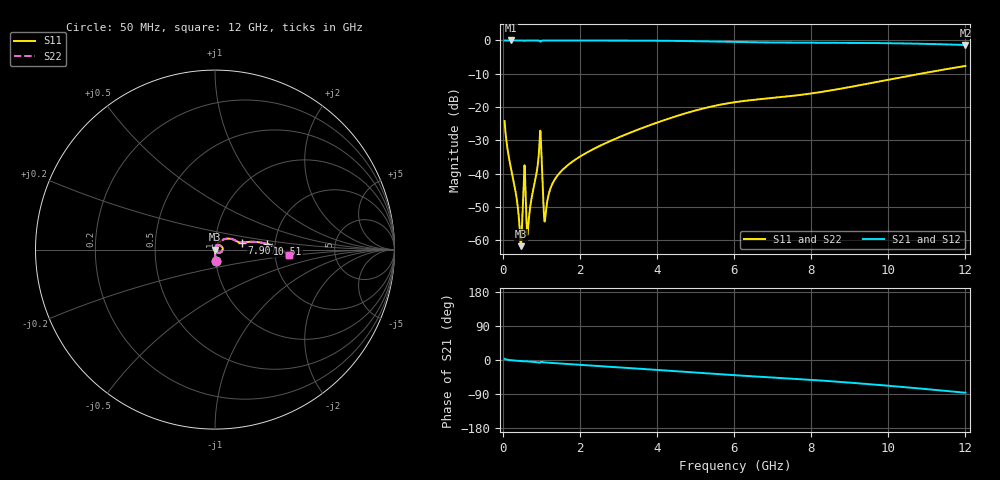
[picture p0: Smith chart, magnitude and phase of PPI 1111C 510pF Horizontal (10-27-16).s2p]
# MHz S MA R 50
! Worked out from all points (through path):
!   1601 points, 50 MHz to 12 GHz, reference 50 ohm
!   highest |S21| = 0.00 dB at 214.3 MHz (marker M1); lowest = -1.4 dB at 12 GHz (marker M2)
!   group delay of S21, straight-line fit = 19.5 ps
!   lowest |S11| = -61.8 dB at 475.7 MHz (marker M3), VSWR 1.00, Z = 50.1 + j0.00375 ohm
!   |S11| at or under -10 dB: start of sweep to 10.84 GHz
!   |S22| runs from -61.8 to -7.7 dB; largest |S21 - S12| = 0
!   S11 on the Smith chart (normalised r, x): 50 MHz: 1.00, -0.12; 7.907 GHz: 1.35, +0.11; 10.51 GHz: 1.81, +0.12; 12 GHz: 2.39, -0.19
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50  0.06142 -86.5  0.9978 3.2  0.9978 3.2  0.06142 -86.5
214.3125  0.01205 -88.3  0.9994 -0.6  0.9994 -0.6  0.01205 -88.3
348.75  0.00476 -84.8  0.9994 -1.8  0.9994 -1.8  0.00476 -84.8
430.9062  0.001803 -70.2  0.9993 -2.4  0.9993 -2.4  0.001803 -70.2
475.7188  0.0008118 2.6  0.9992 -2.8  0.9992 -2.8  0.0008118 2.6
557.875  0.01054 38.3  0.9921 -3.6  0.9921 -3.6  0.01054 38.3
647.5  0.001256 22.7  0.9988 -3.8  0.9988 -3.8  0.001256 22.7
677.375  0.002032 56.4  0.999 -4.0  0.999 -4.0  0.002032 56.4
953.7188  0.02735 56.0  0.9872 -6.9  0.9872 -6.9  0.02735 56.0
991.0625  0.03131 -35.6  0.9729 -4.8  0.9729 -4.8  0.03131 -35.6
1065.75  0.00269 -35.8  0.9976 -6.1  0.9976 -6.1  0.00269 -35.8
1110.562  0.002342 40.6  0.9983 -6.5  0.9983 -6.5  0.002342 40.6
1237.531  0.005942 71.1  0.9987 -7.5  0.9987 -7.5  0.005942 71.1
1379.438  0.008646 74.0  0.9987 -8.5  0.9987 -8.5  0.008646 74.0
2044.156  0.01858 72.7  0.9983 -12.9  0.9983 -12.9  0.01858 72.7
4038.312  0.05927 56.0  0.9902 -26.5  0.9902 -26.5  0.05927 56.0
6025  0.1182 27.7  0.9491 -40.1  0.9491 -40.1  0.1182 27.7
7907.125  0.157 14.6  0.9261 -51.7  0.9261 -51.7  0.157 14.6
8019.156  0.1603 14.4  0.9257 -52.5  0.9257 -52.5  0.1603 14.4
10013.31  0.2574 8.8  0.909 -68.0  0.909 -68.0  0.2574 8.8
10506.25  0.2915 6.2  0.8998 -72.4  0.8998 -72.4  0.2915 6.2
12000  0.4136 -4.5  0.854 -86.4  0.854 -86.4  0.4136 -4.5
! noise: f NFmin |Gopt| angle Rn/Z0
50  0.0003593  0.8616  0.33  0.0005564
1372  0.003857  0.6817  7.924  0.002335
2701  0.007523  0.6824  15.46  0.004509
4031  0.01691  0.7811  22.94  0.01522
5360  0.03712  0.8647  30.24  0.05493
6682  0.05881  0.8952  37.22  0.11
8012  0.06672  0.8934  43.92  0.1174
9341  0.06911  0.8853  50.29  0.1073
1.067e+04  0.07194  0.88  56.33  0.1009
1.2e+04  0.07625  0.8786  62.02  0.09996
